INTERFACE I_ApplicationState

PROPERTY PUBLIC CurrentState : I_Substate
GET
END_GET
END_PROPERTY

METHOD PUBLIC MoveNext : BOOL
VAR_INPUT
END_VAR
END_METHOD

METHOD PUBLIC Reset
VAR_INPUT
END_VAR
END_METHOD

END_INTERFACE
